|   IBIS file stm32l471_475_476_486_lqfp64.ibs
[IBIS ver]   4.2
[File name]   stm32l471_475_476_486_lqfp64.ibs
[File Rev]   4.0
[Date]   08-10-2018
[Source]   Data Created at STMicroelectronics
[Notes]   File originated from ELDO simulations.
[Disclaimer]  This information is for modeling purpose only and is
   not guaranteed.
   The information is subject to change without notice.
[Copyright]   Copyright 2018 STMicroelectronics Inc.
|   Component stm32l471_475_476_486_lqfp64
[Component] stm32l471_475_476_486_lqfp64
[Manufacturer] STMicroelectronics
[Package]
| variable   typ   min   max
R_pkg   0.0   0.0   0.0
L_pkg   0.0H   0.0H   0.0H
C_pkg   0.0F   0.0F   0.0F
[Pin]  signal_name   model_name   R_pin   L_pin   C_pin
1 VBAT POWER 68.980E-3 4.220E-9 120.000E-15
2 PC13 io8prog2m25m50m120m_sudq_ft 63.756E-3 3.679E-9 93.469E-15
3 PC14-OSC32_IN io8prog2m25m50m120m_sudq_ft 59.336E-3 3.221E-9 71.020E-15
4 PC15-OSC32_OUT io8prog2m25m50m120m_sudq_ft 55.719E-3 2.846E-9 52.653E-15
5 PH0-OSC_IN io8prog2m25m50m120m_sudq_ft 52.907E-3 2.555E-9 38.367E-15
6 PH1-OSC_OUT io8prog2m25m50m120m_sudq_ft 50.897E-3 2.347E-9 28.163E-15
7 NRST ioreset_ft_v33 49.692E-3 2.222E-9 22.041E-15
8 PC0 io8prog2m25m50m120m_sudq_i2c_ft 49.290E-3 2.180E-9 20.000E-15
9 PC1 io8prog2m25m50m120m_sudq_i2c_ft 49.290E-3 2.180E-9 20.000E-15
10 PC2 io8prog2m25m50m120m_sudq_ft 49.692E-3 2.222E-9 22.041E-15
11 PC3 io8prog2m25m50m120m_sudq_ft 50.897E-3 2.347E-9 28.163E-15
12 VSSA/VREF- GND 52.907E-3 2.555E-9 38.367E-15
13 VDDA/VREF+ POWER 55.719E-3 2.846E-9 52.653E-15
14 PA0 io8prog2m25m50m120m_sudq_ft 59.336E-3 3.221E-9 71.020E-15
15 PA1 io8prog2m25m50m120m_sudq_ft 63.756E-3 3.679E-9 93.469E-15
16 PA2 io8prog2m25m50m120m_sudq_ft 68.980E-3 4.220E-9 120.000E-15
17 PA3 io8prog2m25m50m120m_sudq_ft 68.980E-3 4.220E-9 120.000E-15
18 VSS GND 63.756E-3 3.679E-9 93.469E-15
19 VDD POWER 59.336E-3 3.221E-9 71.020E-15
20 PA4 io8prog2m25m50m120m_sudq_ft 55.719E-3 2.846E-9 52.653E-15
21 PA5 io8prog2m25m50m120m_sudq_ft 52.907E-3 2.555E-9 38.367E-15
22 PA6 io8prog2m25m50m120m_sudq_ft 50.897E-3 2.347E-9 28.163E-15
23 PA7 io8prog2m25m50m120m_sudq_ft 49.692E-3 2.222E-9 22.041E-15
24 PC4 io8prog2m25m50m120m_sudq_ft 49.290E-3 2.180E-9 20.000E-15
25 PC5 io8prog2m25m50m120m_sudq_ft 49.290E-3 2.180E-9 20.000E-15
26 PB0 io8prog2m25m50m120m_sudq_ft 49.692E-3 2.222E-9 22.041E-15
27 PB1 io8prog2m25m50m120m_sudq_ft 50.897E-3 2.347E-9 28.163E-15
28 PB2 io8prog2m25m50m120m_sudq_ft 52.907E-3 2.555E-9 38.367E-15
29 PB10 io8prog2m25m50m120m_sudq_i2c_ft 55.719E-3 2.846E-9 52.653E-15
30 PB11 io8prog2m25m50m120m_sudq_i2c_ft 59.336E-3 3.221E-9 71.020E-15
31 VSS GND 63.756E-3 3.679E-9 93.469E-15
32 VDD POWER 68.980E-3 4.220E-9 120.000E-15
33 PB12 io8w_swp_lcd4_ft 68.980E-3 4.220E-9 120.000E-15
34 PB13 io8prog2m25m50m120m_sudq_i2c_ft 63.756E-3 3.679E-9 93.469E-15
35 PB14 io8prog2m25m50m120m_sudq_i2c_ft 59.336E-3 3.221E-9 71.020E-15
36 PB15 io8prog2m25m50m120m_sudq_ft 55.719E-3 2.846E-9 52.653E-15
37 PC6 io8prog2m25m50m120m_sudq_ft 52.907E-3 2.555E-9 38.367E-15
38 PC7 io8prog2m25m50m120m_sudq_ft 50.897E-3 2.347E-9 28.163E-15
39 PC8 io8prog2m25m50m120m_sudq_ft 49.692E-3 2.222E-9 22.041E-15
40 PC9 io8prog2m25m50m120m_sudq_ft 49.290E-3 2.180E-9 20.000E-15
41 PA8 io8prog2m25m50m120m_sudq_ft 49.290E-3 2.180E-9 20.000E-15
42 PA9 POWER 49.692E-3 2.222E-9 22.041E-15
43 PA10 io8usb_id_otg20_lcd4_ft_ms 50.897E-3 2.347E-9 28.163E-15
44 PA11 io8usblsfs_otg2 52.907E-3 2.555E-9 38.367E-15
45 PA12 io8usblsfs_otg2 55.719E-3 2.846E-9 52.653E-15
46 PA13 io8prog2m25m50m120m_sudq_ft 59.336E-3 3.221E-9 71.020E-15
47 VSS GND 63.756E-3 3.679E-9 93.469E-15
48 VDDUSB/VDD POWER 68.980E-3 4.220E-9 120.000E-15
49 PA14 io8prog2m25m50m120m_sudq_ft 68.980E-3 4.220E-9 120.000E-15
50 PA15 io8prog2m25m50m120m_sudq_ft 63.756E-3 3.679E-9 93.469E-15
51 PC10 io8prog2m25m50m120m_sudq_ft 59.336E-3 3.221E-9 71.020E-15
52 PC11 io8prog2m25m50m120m_sudq_ft 55.719E-3 2.846E-9 52.653E-15
53 PC12 io8prog2m25m50m120m_sudq_ft 52.907E-3 2.555E-9 38.367E-15
54 PD2 io8prog2m25m50m120m_sudq_ft 50.897E-3 2.347E-9 28.163E-15
55 PB3 io8prog2m25m50m120m_sudq_ft 49.692E-3 2.222E-9 22.041E-15
56 PB4 io8prog2m25m50m120m_sudq_ft 49.290E-3 2.180E-9 20.000E-15
57 PB5 io8prog2m25m50m120m_sudq_ft 49.290E-3 2.180E-9 20.000E-15
58 PB6 io8prog2m25m50m120m_sudq_i2c_ft 49.692E-3 2.222E-9 22.041E-15
59 PB7 io8prog2m25m50m120m_sudq_i2c_ft 50.897E-3 2.347E-9 28.163E-15
60 BOOT0 vpp_test_hv 52.907E-3 2.555E-9 38.367E-15
61 PB8 io8prog2m25m50m120m_sudq_i2c_ft 55.719E-3 2.846E-9 52.653E-15
62 PB9 io8prog2m25m50m120m_sudq_i2c_ft 59.336E-3 3.221E-9 71.020E-15
63 VSS GND 63.756E-3 3.679E-9 93.469E-15
64 VDD POWER 68.980E-3 4.220E-9 120.000E-15
[Model Selector] io8prog2m25m50m120m_sudq_ft
iols8p_sudq_ft_pd_lv  "IO low speed, PD=40kOhm - 1P8V"
iols8p_sudq_ft_pu_lv  "IO low speed, PU=40kOhm - 1P8V"
iols8p_sudq_ft_lv  "IO low speed - 1P8V"
iols8p_sudq_ft_pd  "IO low speed, PD=40kOhm - 3P3V"
iols8p_sudq_ft_pu  "IO low speed, PU=40kOhm - 3P3V"
iols8p_sudq_ft  "IO low speed - 3P3V"
iofs8p_sudq_ft_pd_lv  "IO full speed, PD=40kOhm - 1P8V"
iofs8p_sudq_ft_pu_lv  "IO full speed, PU=40kOhm - 1P8V"
iofs8p_sudq_ft_lv  "IO full speed - 1P8V"
iofs8p_sudq_ft_pd  "IO full speed, PD=40kOhm - 3P3V"
iofs8p_sudq_ft_pu  "IO full speed, PU=40kOhm - 3P3V"
iofs8p_sudq_ft  "IO full speed - 3P3V"
ioms8p_sudq_ft_pd_lv  "IO medium speed, PD=40kOhm - 1P8V"
ioms8p_sudq_ft_pu_lv  "IO medium speed, PU=40kOhm - 1P8V"
ioms8p_sudq_ft_lv  "IO medium speed - 1P8V"
ioms8p_sudq_ft_pd  "IO medium speed, PD=40kOhm - 3P3V"
ioms8p_sudq_ft_pu  "IO medium speed, PU=40kOhm - 3P3V"
ioms8p_sudq_ft  "IO medium speed - 3P3V"
iohs8p_sudq_ft_pd_lv  "IO high speed, PD=40kOhm - 1P8V"
iohs8p_sudq_ft_pu_lv  "IO high speed, PU=40kOhm - 1P8V"
iohs8p_sudq_ft_lv  "IO high speed - 1P8V"
iohs8p_sudq_ft_pd  "IO high speed, PD=40kOhm - 3P3V"
iohs8p_sudq_ft_pu  "IO high speed, PU=40kOhm - 3P3V"
iohs8p_sudq_ft  "IO high speed - 3P3V"
[Model Selector] io8prog2m25m50m120m_sudq_i2c_ft
io8prog_1v8_i2c_pd  "5V Tol GPIO 1.8V range i2c functionality with pull down"
io8prog_1v8_i2c_pu  "5V Tol GPIO 1.8V range i2c functionality with pull up"
io8prog_1v8_i2c  "5V Tol GPIO 1.8V range i2c functionality"
io8prog_3v3_i2c_pd  "5V Tol GPIO 3.3V range i2c functionality with pull down"
io8prog_3v3_i2c_pu  "5V Tol GPIO 3.3V range i2c functionality with pull up"
io8prog_3v3_i2c  "5V Tol GPIO 3.3V range i2c functionality"
io8ls_1v8_pd  "5V Tol GPIO 1.8V range with pd io low speed"
io8ls_1v8_pu  "5V Tol GPIO 1.8V range with pu io low speed"
io8ls_1v8  "5V Tol GPIO 1.8V range io low speed"
io8ls_3v3_pd  "5V Tol GPIO 3.3V range with pd io low speed"
io8ls_3v3_pu  "5V Tol GPIO 3.3V range with pu io low speed"
io8ls_3v3  "5V Tol GPIO 3.3V range io low speed"
io8fs_1v8_pd  "5V Tol GPIO 1.8V range with pd io full speed"
io8fs_1v8_pu  "5V Tol GPIO 1.8V range with pu io full speed"
io8fs_1v8  "5V Tol GPIO 1.8V range io full speed"
io8fs_3v3_pd  "5V Tol GPIO 3.3V range with pd io full speed"
io8fs_3v3_pu  "5V Tol GPIO 3.3V range with pu io full speed"
io8fs_3v3  "5V Tol GPIO 3.3V range io full speed"
io8ms_1v8_pd  "5V Tol GPIO 1.8V range with pd io medium speed"
io8ms_1v8_pu  "5V Tol GPIO 1.8V range with pu io medium speed"
io8ms_1v8  "5V Tol GPIO 1.8V range io medium speed"
io8ms_3v3_pd  "5V Tol GPIO 3.3V range with pd io medium speed"
io8ms_3v3_pu  "5V Tol GPIO 3.3V range with pu io medium speed"
io8ms_3v3  "5V Tol GPIO 3.3V range io medium speed"
io8hs_1v8_pd  "5V Tol GPIO 1.8V range with pd io high speed"
io8hs_1v8_pu  "5V Tol GPIO 1.8V range with pu io high speed"
io8hs_1v8  "5V Tol GPIO 1.8V range io high speed"
io8hs_3v3_pd  "5V Tol GPIO 3.3V range with pd io high speed"
io8hs_3v3_pu  "5V Tol GPIO 3.3V range with pu io high speed"
io8hs_3v3  "5V Tol GPIO 3.3V range io high speed"
[Model Selector] io8usb_id_otg20_lcd4_ft_ms
io8usbid_1v8_id_pu  "ID 1V8 range with pull up"
io8usbid_3v3_id_pu  "ID 3V3 range with pull up"
io8usbid_1v8_id  "ID 1V8 range"
io8usbid_3v3_id  "ID 3V3 range"
io8lsusbid_1v8_pd  "GPIO 1.8V range with pd io low speed"
io8lsusbid_1v8_pu  "GPIO 1.8V range with pu io low speed"
io8lsusbid_1v8  "GPIO 1.8V range io low speed"
io8lsusbid_3v3_pd  "GPIO 3.3V range with pd io low speed"
io8lsusbid_3v3_pu  "GPIO 3.3V range with pu io low speed"
io8lsusbid_3v3  "GPIO 3.3V range io low speed"
io8fsusbid_1v8_pd  "GPIO 1.8V range with pd io full speed"
io8fsusbid_1v8_pu  "GPIO 1.8V range with pu io full speed"
io8fsusbid_1v8  "GPIO 1.8V range io full speed"
io8fsusbid_3v3_pd  "GPIO 3.3V range with pd io full speed"
io8fsusbid_3v3_pu  "GPIO 3.3V range with pu io full speed"
io8fsusbid_3v3  "GPIO 3.3V range io full speed"
io8msusbid_1v8_pd  "GPIO 1.8V range with pd io medium speed"
io8msusbid_1v8_pu  "GPIO 1.8V range with pu io medium speed"
io8msusbid_1v8  "GPIO 1.8V range io medium speed"
io8msusbid_3v3_pd  "GPIO 3.3V range with pd io medium speed"
io8msusbid_3v3_pu  "GPIO 3.3V range with pu io medium speed"
io8msusbid_3v3  "GPIO 3.3V range io medium speed"
io8hsusbid_1v8_pd  "GPIO 1.8V range with pd io high speed"
io8hsusbid_1v8_pu  "GPIO 1.8V range with pu io high speed"
io8hsusbid_1v8  "GPIO 1.8V range io high speed"
io8hsusbid_3v3_pd  "GPIO 3.3V range with pd io high speed"
io8hsusbid_3v3_pu  "GPIO 3.3V range with pu io high speed"
io8hsusbid_3v3  "GPIO 3.3V range io high speed"
[Model Selector] io8usblsfs_otg2
usb_ls_pd  "USB Low Speed mode - Pull Down"
usb_ls_pu2  "USB Low Speed mode - Pull up 2"
usb_ls_pu  "USB Low Speed mode - Pull up"
usb_fs  "USB Low Speed mode"
usb_fs_pd  "USB Full Speed mode - Pull Down"
usb_fs_pu2  "USB Full Speed mode - Pull up 2"
usb_fs_pu  "USB Full Speed mode - Pull up"
[Model Selector] ioreset_ft_v33
ioreset_1v2_pu  "RESET 1.2V range with PU"
ioreset_1v2  "RESET 1.2V range"
ioreset_1v8_pu  "RESET 1.8V range with PU"
ioreset_1v8  "RESET 1.8V range"
ioreset_3v3_pu  "RESET 3.3V range with PU"
ioreset_3v3  "RESET 3.3V range"
[Model Selector] io8w_swp_lcd4_ft
io8w_swp_classc  "Class C swp functionality"
io8w_swp_classb  "Class B swp functionality"
io8lsw_1v8_pd  "GPIO 1.8V range with pd io low speed"
io8lsw_1v8_pu  "GPIO 1.8V range with pu io low speed"
io8lsw_1v8  "GPIO 1.8V range io low speed"
io8lsw_3v3_pd  "GPIO 3.3V range with pd io low speed"
io8lsw_3v3_pu  "GPIO 3.3V range with pu io low speed"
io8lsw_3v3  "GPIO 3.3V range io low speed"
io8fsw_1v8_pd  "GPIO 1.8V range with pd io full speed"
io8fsw_1v8_pu  "GPIO 1.8V range with pu io full speed"
io8fsw_1v8  "GPIO 1.8V range io full speed"
io8fsw_3v3_pd  "GPIO 3.3V range with pd io full speed"
io8fsw_3v3_pu  "GPIO 3.3V range with pu io full speed"
io8fsw_3v3  "GPIO 3.3V range io full speed"
io8msw_1v8_pd  "GPIO 1.8V range with pd io medium speed"
io8msw_1v8_pu  "GPIO 1.8V range with pu io medium speed"
io8msw_1v8  "GPIO 1.8V range io medium speed"
io8msw_3v3_pd  "GPIO 3.3V range with pd io medium speed"
io8msw_3v3_pu  "GPIO 3.3V range with pu io medium speed"
io8msw_3v3  "GPIO 3.3V range io medium speed"
io8hsw_1v8_pd  "GPIO 1.8V range with pd io high speed"
io8hsw_1v8_pu  "GPIO 1.8V range with pu io high speed"
io8hsw_1v8  "GPIO 1.8V range io high speed"
io8hsw_3v3_pd  "GPIO 3.3V range with pd io high speed"
io8hsw_3v3_pu  "GPIO 3.3V range with pu io high speed"
io8hsw_3v3  "GPIO 3.3V range io high speed"
[Model Selector] vpp_test_hv
vpp_1v8  "VPP with test functionality 1.8V range"
vpp_3v3  "VPP with test functionality 3.3V range"
| Models and submodels in the file (123): iols8p_sudq_ft_pd_lv (I/O), iols8p_sudq_ft_pu_lv (I/O), iols8p_sudq_ft_lv (I/O), iols8p_sudq_ft_pd (I/O), iols8p_sudq_ft_pu (I/O), iols8p_sudq_ft (I/O), iofs8p_sudq_ft_pd_lv (I/O), iofs8p_sudq_ft_pu_lv (I/O), iofs8p_sudq_ft_lv (I/O), iofs8p_sudq_ft_pd (I/O), iofs8p_sudq_ft_pu (I/O), iofs8p_sudq_ft (I/O), ioms8p_sudq_ft_pd_lv (I/O), ioms8p_sudq_ft_pu_lv (I/O), ioms8p_sudq_ft_lv (I/O), ioms8p_sudq_ft_pd (I/O), ioms8p_sudq_ft_pu (I/O), ioms8p_sudq_ft (I/O), iohs8p_sudq_ft_pd_lv (I/O), iohs8p_sudq_ft_pu_lv (I/O), iohs8p_sudq_ft_lv (I/O), iohs8p_sudq_ft_pd (I/O), iohs8p_sudq_ft_pu (I/O), iohs8p_sudq_ft (I/O), io8prog_1v8_i2c_pd (I/O), io8prog_1v8_i2c_pu (I/O), io8prog_1v8_i2c (I/O), io8prog_3v3_i2c_pd (I/O), io8prog_3v3_i2c_pu (I/O), io8prog_3v3_i2c (I/O), io8ls_1v8_pd (I/O), io8ls_1v8_pu (I/O), io8ls_1v8 (I/O), io8ls_3v3_pd (I/O), io8ls_3v3_pu (I/O), io8ls_3v3 (I/O), io8fs_1v8_pd (I/O), io8fs_1v8_pu (I/O), io8fs_1v8 (I/O), io8fs_3v3_pd (I/O), io8fs_3v3_pu (I/O), io8fs_3v3 (I/O), io8ms_1v8_pd (I/O), io8ms_1v8_pu (I/O), io8ms_1v8 (I/O), io8ms_3v3_pd (I/O), io8ms_3v3_pu (I/O), io8ms_3v3 (I/O), io8hs_1v8_pd (I/O), io8hs_1v8_pu (I/O), io8hs_1v8 (I/O), io8hs_3v3_pd (I/O), io8hs_3v3_pu (I/O), io8hs_3v3 (I/O), io8usbid_1v8_id_pu (Input), io8usbid_3v3_id_pu (Input), io8usbid_1v8_id (Input), io8usbid_3v3_id (Input), io8lsusbid_1v8_pd (I/O), io8lsusbid_1v8_pu (I/O), io8lsusbid_1v8 (I/O), io8lsusbid_3v3_pd (I/O), io8lsusbid_3v3_pu (I/O), io8lsusbid_3v3 (I/O), io8fsusbid_1v8_pd (I/O), io8fsusbid_1v8_pu (I/O), io8fsusbid_1v8 (I/O), io8fsusbid_3v3_pd (I/O), io8fsusbid_3v3_pu (I/O), io8fsusbid_3v3 (I/O), io8msusbid_1v8_pd (I/O), io8msusbid_1v8_pu (I/O), io8msusbid_1v8 (I/O), io8msusbid_3v3_pd (I/O), io8msusbid_3v3_pu (I/O), io8msusbid_3v3 (I/O), io8hsusbid_1v8_pd (I/O), io8hsusbid_1v8_pu (I/O), io8hsusbid_1v8 (I/O), io8hsusbid_3v3_pd (I/O)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
